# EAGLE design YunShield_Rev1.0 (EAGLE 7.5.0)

## Sheet 1 of 2: MAIN SCHEMATIC
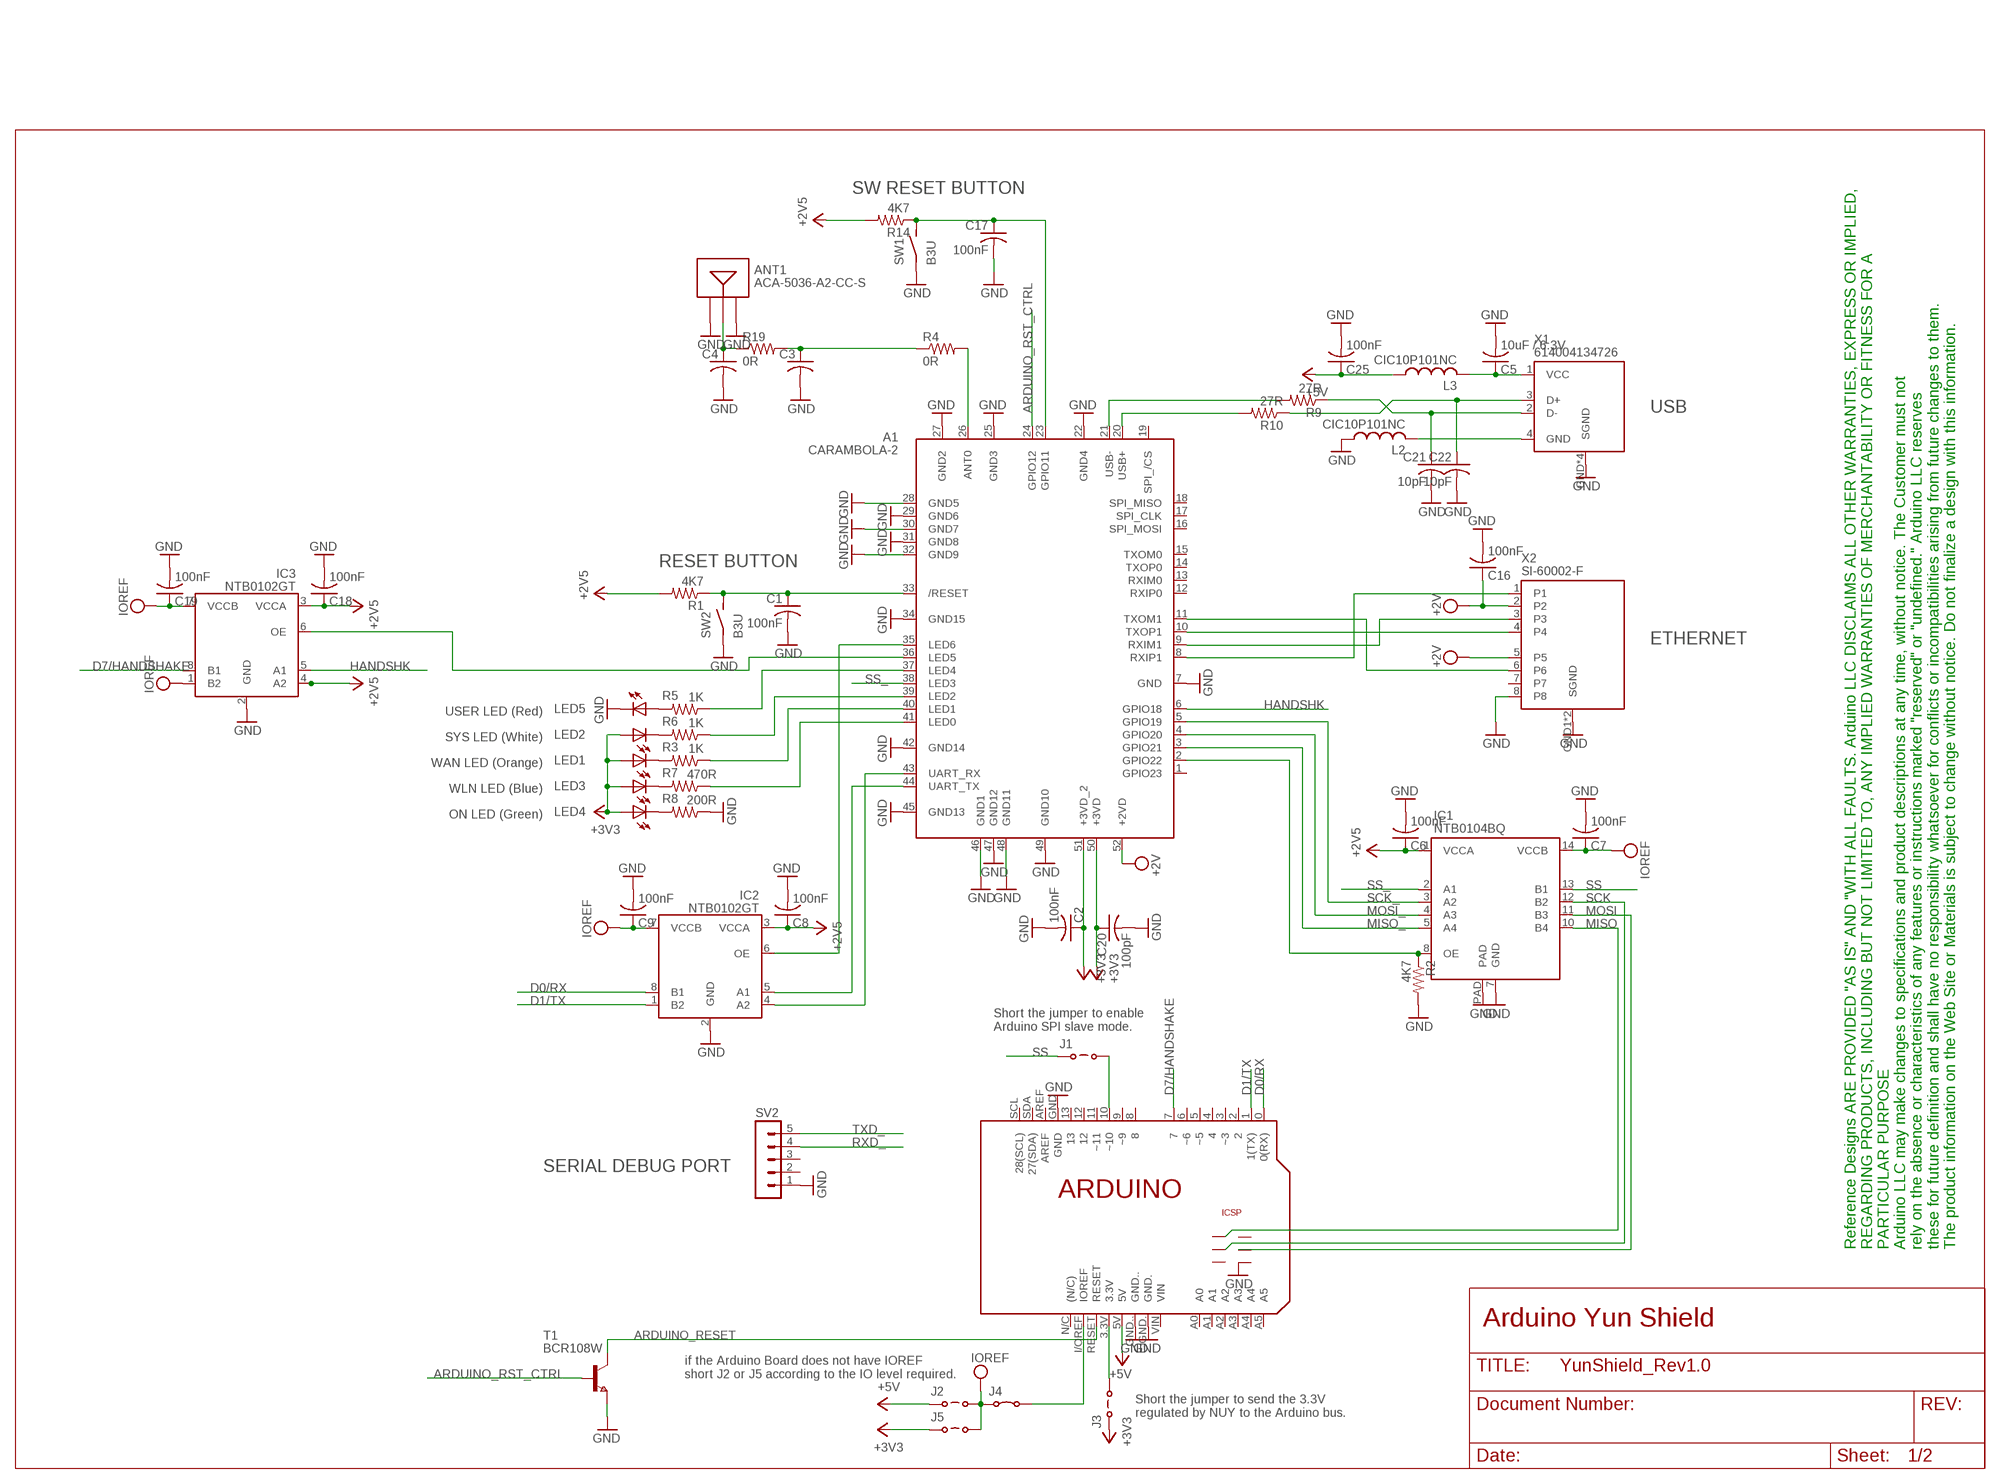
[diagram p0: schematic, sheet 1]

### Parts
A1  CARAMBOLA-2  [CARAMBOLA-2]
ANT1  ACA-5036-A2-CC-S  [ACA-5036-A2-CC-S]
C1  100nF  C-USC0402  [C0402]
C2  100nF  C-USC0402  [C0402]
C3  C-USC0402  [C0402]
C4  C-USC0402  [C0402]
C5  10uF / 6.3V  C-USC1608  [C1608]
C6  100nF  C-USC0402  [C0402]
C7  100nF  C-USC0402  [C0402]
C8  100nF  C-USC0402  [C0402]
C9  100nF  C-USC0402  [C0402]
C16  100nF  C-USC0402  [C0402]
C17  100nF  C-USC0402  [C0402]
C18  100nF  C-USC0402  [C0402]
C19  100nF  C-USC0402  [C0402]
C20  100pF  C-USC0402  [C0402]
C21  10pF  C-USC0402  [C0402]
C22  10pF  C-USC0402  [C0402]
C25  100nF  C-USC0402  [C0402]
IC1  NTB0104BQ  [DHVQFN14]
IC2  NTB0102GT  [XSON8]
IC3  NTB0102GT  [XSON8]
J1  JUMPER-OPEN  [JUMPER-OPEN]
J2  JUMPER-OPEN  [JUMPER-OPEN]
J3  JUMPER-OPEN  [JUMPER-OPEN]
J4  JUMPER-CLOSED  [JUMPER-CLOSED]
J5  JUMPER-OPEN  [JUMPER-OPEN]
L2  CIC10P101NC  L-US  [R0603]
L3  CIC10P101NC  L-US  [R0603]
LED1  LTST-C191KFKT  LEDCHIP-LED0603  [CHIP-LED0603]
LED2  LTW-C193TS5  LEDCHIP-LED0603  [CHIP-LED0603]
LED3  LTST-C191TBKT  LEDCHIP-LED0603  [CHIP-LED0603]
LED4  LTST-C191KGKT  LEDCHIP-LED0603  [CHIP-LED0603]
LED5  LTST-C191KRKT  LEDCHIP-LED0603  [CHIP-LED0603]
PCB1  ARDUINO_UNO  [ARDUINO_UNO]
R1  4K7  R-US_R0402  [R0402]
R2  4K7  R-US_R0402  [R0402]
R3  1K  R-US_R0402  [R0402]
R4  0R  R-US_R0402  [R0402]
R5  1K  R-US_R0402  [R0402]
R6  1K  R-US_R0402  [R0402]
R7  470R  R-US_R0402  [R0402]
R8  200R  R-US_R0402  [R0402]
R9  27R  R-US_R0402  [R0402]
R10  27R  R-US_R0402  [R0402]
R14  4K7  R-US_R0402  [R0402]
R19  0R  R-US_R0402  [R0402]
SV2  MA05-1  [MA05-1]
SW1  B3U  [B3U]
SW2  B3U  [B3U]
T1  BCR108W  NPNSOT323  [SOT323]
X1  614004134726  [614004134726]
X2  SI-60002-F  [SI-60002-F]

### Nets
+3V3: A1.50(+3VD) A1.51(+3VD_2) C2.1 C20.1 J3.1 J5.1 LED1.A LED2.A LED3.A LED4.A ; also sheet 2
+5V: C25.1 J2.1 L3.1 PCB1.5V ; also sheet 2
ARDUINO_RESET: PCB1.RESET T1.1(C)
ARDUINO_RST_CTRL: A1.24(GPIO12) T1.2(B)
D0/RX: IC2.8(B1) PCB1.0(0(RX))
D1/TX: IC2.1(B2) PCB1.1(1(TX))
D7/HANDSHAKE: IC3.8(B1) PCB1.7
GND: A1.7(GND) A1.22(GND4) A1.25(GND3) A1.27(GND2) A1.28(GND5) A1.29(GND6) A1.30(GND7) A1.31(GND8) A1.32(GND9) A1.34(GND15) A1.42(GND14) A1.45(GND13) A1.46(GND1) A1.47(GND12) A1.48(GND11) A1.49(GND10) ANT1.GND ANT1.GND2 C1.2 C2.2 C3.2 C4.2 C5.2 C6.2 C7.2 C8.2 C9.2 C16.2 C17.2 C18.2 C19.2 C20.2 C21.2 C22.2 C25.2 IC1.7(GND) IC1.PAD IC2.2(GND) IC3.2(GND) L2.1 LED5.C PCB1.GND PCB1.GND. PCB1.GND.. PCB1.GND_ R2.2 R8.1 SV2.1 SW1.1 SW2.1 T1.3(E) X1.GND1(SGND) X1.GND2(SGND) X1.GND3(SGND) X1.GND(SGND) X2.8 X2.GND1(SGND) X2.GND2(SGND) ; also sheet 2
HANDSHK: A1.6(GPIO18) IC3.5(A1)
MISO: IC1.10(B4) PCB1.MISO
MISO_: A1.3(GPIO21) IC1.5(A4)
MOSI: IC1.11(B3) PCB1.MOSI
MOSI_: A1.4(GPIO20) IC1.4(A3)
N$1: A1.40(LED1) R3.1
N$2: A1.20(USB+) R10.2
N$3: A1.21(USB-) R9.2
N$4: C5.1 L3.2 X1.1(VCC)
N$5: LED1.C R3.2
N$6: L2.2 X1.4(GND)
N$7: J1.2 PCB1.10(~10)
N$8: J3.2 PCB1.3.3V
N$9: LED5.A R5.2
N$10: C3.1 R4.1 R19.2
N$11: A1.2(GPIO22) IC1.8(OE) R2.1
N$12: A1.37(LED4) R5.1
N$15: LED3.C R7.2
N$16: LED2.C R6.2
N$17: C22.1 R10.1 X1.3(D+)
N$19: A1.23(GPIO11) C17.1 R14.1 SW1.2
N$21: A1.39(LED2) R6.1
N$24: LED4.C R8.2
N$25: A1.41(LED0) R7.1
N$26: A1.35(LED6) IC2.6(OE)
N$27: C21.1 R9.1 X1.2(D-)
N$28: J4.2 PCB1.I/OREF(IOREF)
N$31: A1.36(LED5) IC3.6(OE)
N$33: ANT1.FEED C4.1 R19.1
N$35: A1.26(ANT0) R4.2
N$36: A1.11(TXOM1) X2.6
N$37: A1.10(TXOP1) X2.4
N$38: A1.9(RXIM1) X2.3
N$39: A1.8(RXIP1) X2.1
RESET: A1.33(/RESET) C1.1 R1.1 SW2.2
RXD_: A1.43(UART_RX) IC2.4(A2) SV2.4
SCK: IC1.12(B2) PCB1.SCK
SCK_: A1.5(GPIO19) IC1.3(A2)
SS: IC1.13(B1) J1.1
SS_: A1.38(LED3) IC1.2(A1)
TXD_: A1.44(UART_TX) IC2.5(A1) SV2.5
V+: C6.1 C8.1 C18.1 IC1.1(VCCA) IC2.3(VCCA) IC3.3(VCCA) IC3.4(A2) R1.2 R14.2 ; supply symbol labelled +2V5 ; also sheet 2
VEE: A1.52(+2VD) C16.1 X2.2 X2.5 ; supply symbol labelled +2V
VPP: C7.1 C9.1 C19.1 IC1.14(VCCB) IC2.7(VCCB) IC3.1(B2) IC3.7(VCCB) J2.2 J4.1 J5.2 ; supply symbol labelled IOREF
Unconnected: A1.1(GPIO23) A1.12(RXIP0) A1.13(RXIM0) A1.14(TXOP0) A1.15(TXOM0) A1.16(SPI_MOSI) A1.17(SPI_CLK) A1.18(SPI_MISO) A1.19(SPI_/CS) PCB1.2 PCB1.3(~3) PCB1.4 PCB1.5(~5) PCB1.6(~6) PCB1.8 PCB1.9(~9) PCB1.11(~11) PCB1.12 PCB1.13 PCB1.+5V PCB1.A0 PCB1.A1 PCB1.A2 PCB1.A3 PCB1.A4 PCB1.A5 PCB1.AREF PCB1.N/C((N/C)) PCB1.RESET. PCB1.SCL(28(SCL)) PCB1.SDA(27(SDA)) PCB1.VIN SV2.2 SV2.3 X2.7

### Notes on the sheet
- SW RESET BUTTON
- USB
- RESET BUTTON
- ETHERNET
- USER LED (Red)
- SYS LED (White)
- WAN LED (Orange)
- WLN LED (Blue)
- ON LED (Green)
- Short the jumper to enable
  Arduino SPI slave mode.
- SERIAL DEBUG PORT
- Reference Designs ARE PROVIDED "AS IS" AND "WITH ALL FAULTS. Arduino LLC DISCLAIMS ALL OTHER WARRANTIES, EXPRESS OR IMPLIED,
  REGARDING PRODUCTS, INCLUDING BUT NOT LIMITED TO, ANY IMPLIED WARRANTIES OF MERCHANTABILITY OR FITNESS FOR A 
  PARTICULAR PURPOSE 
  Arduino LLC may make changes to specifications and product descriptions at any time, without notice. The Customer must not
  rely on the absence or characteristics of any features or instructions marked "reserved" or "undefined." Arduino LLC reserves
  these for future definition and shall have no responsibility whatsoever for conflicts or incompatibilities arising from future changes to them.
  The product information on the Web Site or Materials is subject to change without notice. Do not finalize a design with this information.
- Arduino Yun Shield
- if the Arduino Board does not have IOREF
  short J2 or J5 according to the IO level required.
- Short the jumper to send the 3.3V 
  regulated by NUY to the Arduino bus.

## Sheet 2 of 2: SWITCH-MODE POWER SUPPLY
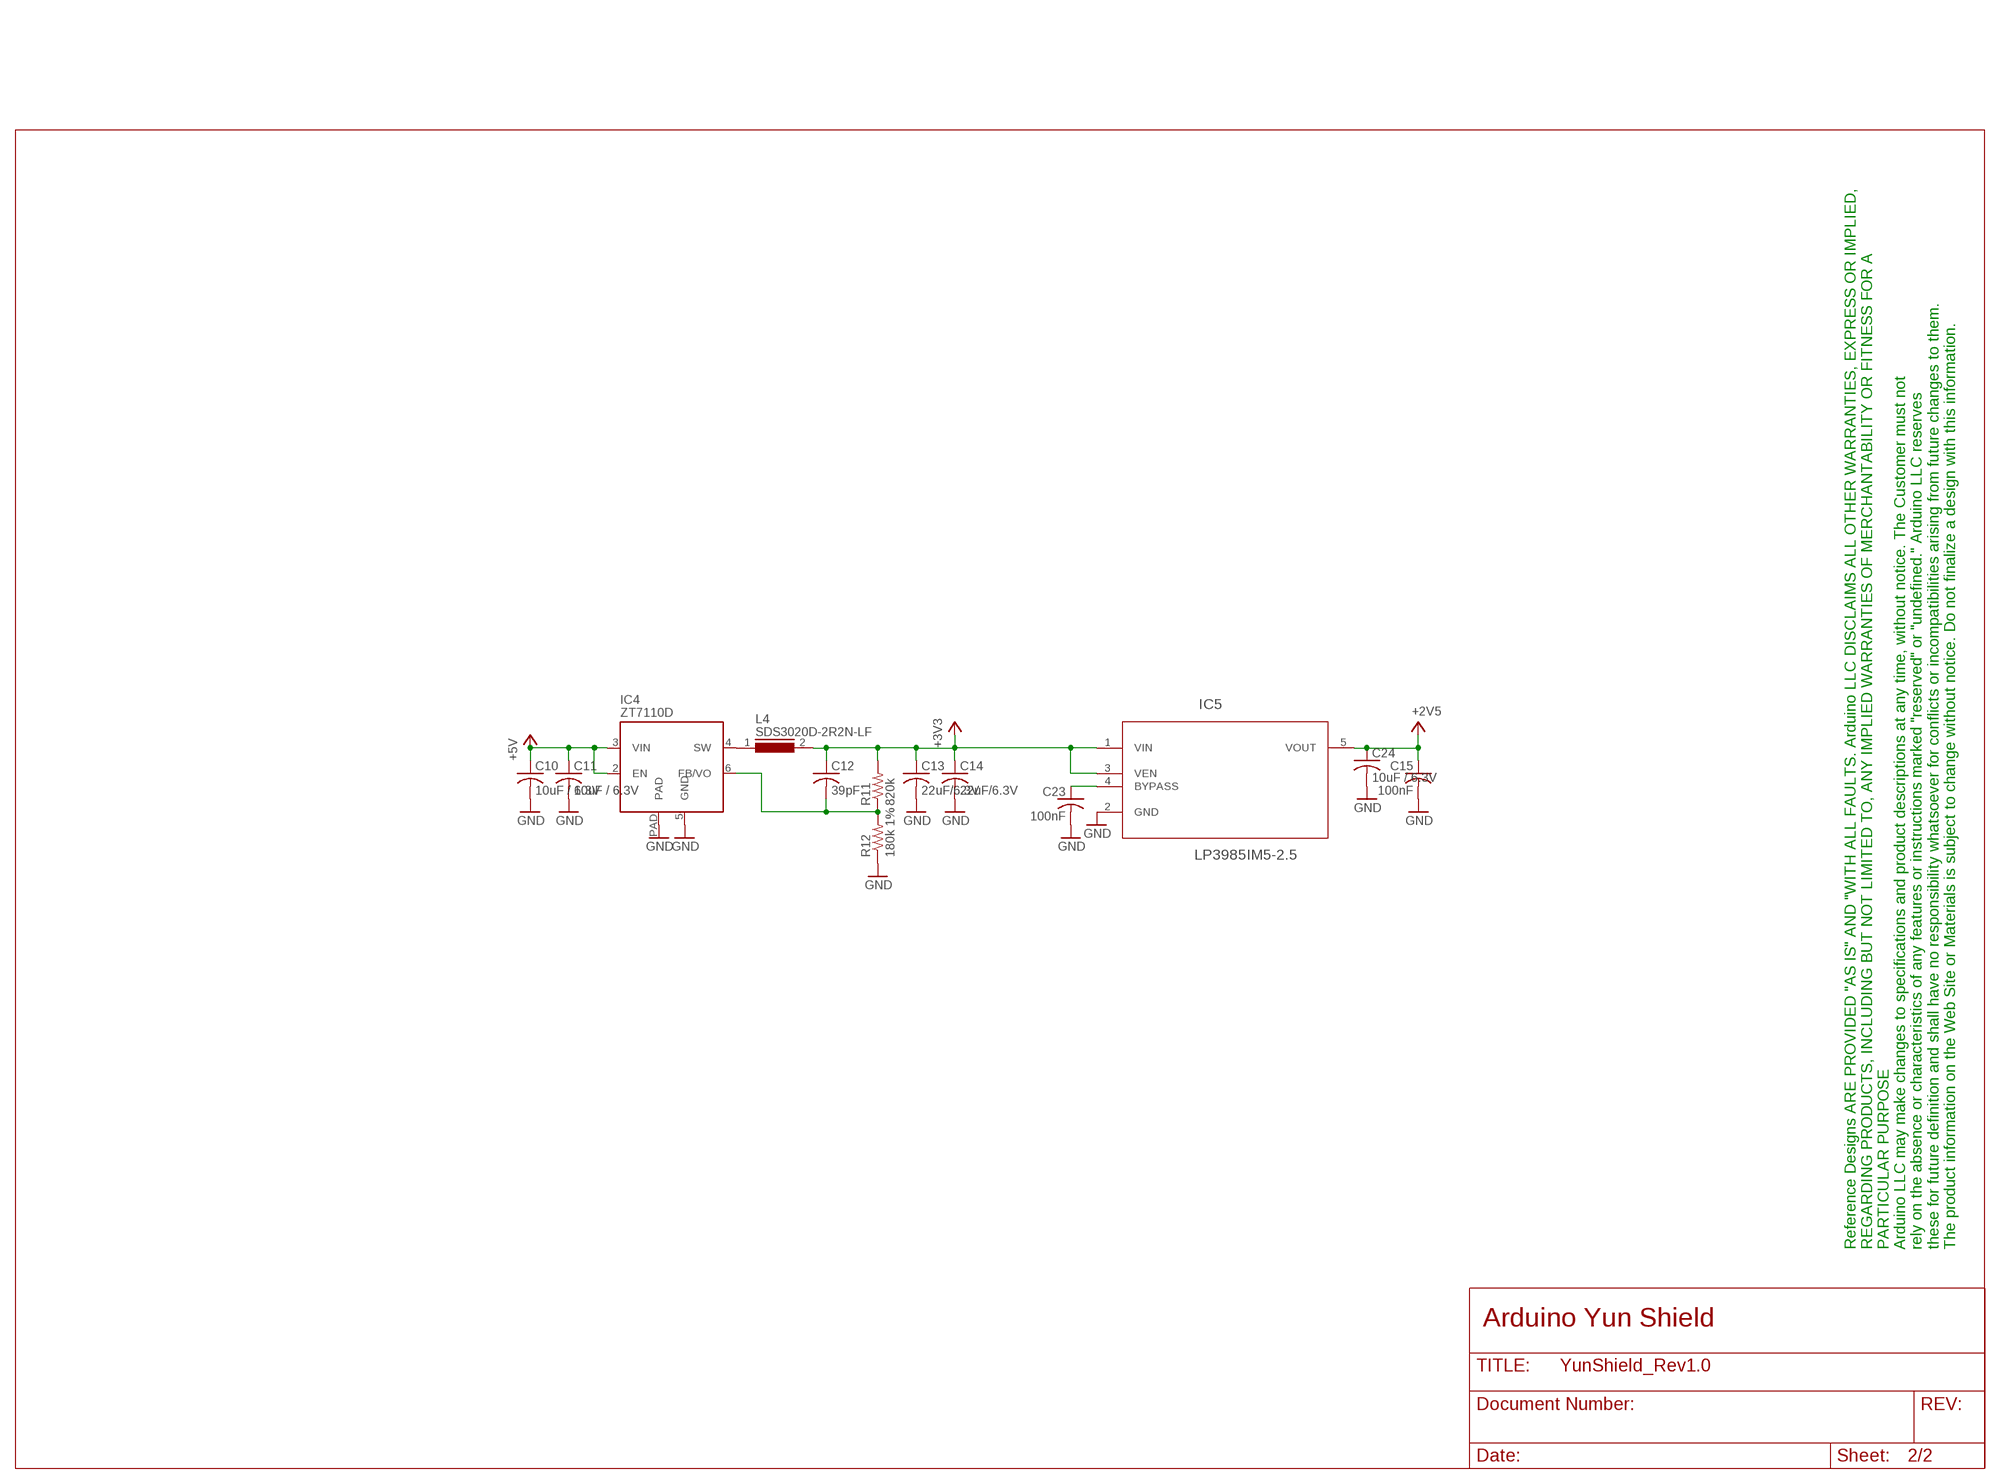
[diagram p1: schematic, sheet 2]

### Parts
C10  10uF / 6.3V  C-USC1608  [C1608]
C11  10uF / 6.3V  C-USC1608  [C1608]
C12  39pF  C-USC0402  [C0402]
C13  22uF/6.3V  C-USC1206  [C1206]
C14  22uF/6.3V  C-USC1206  [C1206]
C15  100nF  C-USC0402  [C0402]
C23  100nF  C-USC0402  [C0402]
C24  10uF / 6.3V  C-USC1608  [C1608]
IC4  ZT7110D  [DFN-6]
IC5  LP3985IM5-2.5  [SOT95P300X120-5N]
L4  SDS3020D-2R2N-LF  [SDS3020D-2R2N-LF]
R11  820k  R-US_R0402  [R0402]
R12  180k 1%  R-US_R0402  [R0402]

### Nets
+3V3: C12.1 C13.1 C14.1 IC5.1(VIN) IC5.3(VEN) L4.2 R11.2 ; also sheet 1
+5V: C10.1 C11.1 IC4.2(EN) IC4.3(VIN) ; also sheet 1
GND: C10.2 C11.2 C13.2 C14.2 C15.2 C23.2 C24.2 IC4.5(GND) IC4.PAD IC5.2(GND) R12.1 ; also sheet 1
N$18: C12.2 IC4.6(FB/VO) R11.1 R12.2
N$20: IC4.4(SW) L4.1
RESET2: C23.1 IC5.4(BYPASS)
V+: C15.1 C24.1 IC5.5(VOUT) ; supply symbol labelled +2V5 ; also sheet 1

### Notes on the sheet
- Reference Designs ARE PROVIDED "AS IS" AND "WITH ALL FAULTS. Arduino LLC DISCLAIMS ALL OTHER WARRANTIES, EXPRESS OR IMPLIED,
  REGARDING PRODUCTS, INCLUDING BUT NOT LIMITED TO, ANY IMPLIED WARRANTIES OF MERCHANTABILITY OR FITNESS FOR A 
  PARTICULAR PURPOSE 
  Arduino LLC may make changes to specifications and product descriptions at any time, without notice. The Customer must not
  rely on the absence or characteristics of any features or instructions marked "reserved" or "undefined." Arduino LLC reserves
  these for future definition and shall have no responsibility whatsoever for conflicts or incompatibilities arising from future changes to them.
  The product information on the Web Site or Materials is subject to change without notice. Do not finalize a design with this information.
- Arduino Yun Shield

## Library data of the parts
A1 = KRB-EX1002-G1413:CARAMBOLA-2
ANT1 = KRB-EX1002-G1413:ACA-5036-A2-CC-S
C1 C3 C4 C6-C9 C15-C19 C21-C23 C25 = KRB-EX1002-G1413:C-US: CAPACITOR, American symbol
C2 C5 C10-C14 C20 C24 = rcl:C-US: CAPACITOR, American symbol
IC1 = KRB-EX1002-G1413:NTB0104
IC2 IC3 = KRB-EX1002-G1413:NTB0102
IC4 = KRB-EX1002-G1413:ZT7110
IC5 = LP3985IM5-2.5:LP3985IM5-2.5: Low-Dropout CMOS Voltage Regulator; MPN: LP3985IM5-25; OC_FARNELL: 1469024; OC_NEWARK: 23K8220; PACKAGE: SOT-5; SIPPLIER: NationalSemiconductor
J1-J3 J5 = rcl:JUMPER-OPEN
J4 = rcl:JUMPER-CLOSED
L2 L3 = rcl:L-US: INDUCTOR, American symbol
L4 = KRB-EX1002-G1413:SDS3020D-2R2N-LF
LED1-LED5 = led:LED: LED
PCB1 = KRB-EX1002-G1413:ARDUINO_UNO: Device for representing an Arduino Uno board with a footprint in an EAGLE design. Created by Dave Young for Element14. More EAGLE documentation at: http://www.element14.com/community/community/knode/cadsoft_eagle
R1-R3 R5-R12 R14 = rcl:R-US_: RESISTOR, American symbol
R4 R19 = KRB-EX1001-G1405:R-US_: RESISTOR, American symbol
SV2 = con-lstb:MA05-1: PIN HEADER; OC_FARNELL: unknown; OC_NEWARK: unknown
SW1 SW2 = 8DEV-1100-0001:B3U
T1 = zetex:NPNSOT323: NPN TRANSISTOR; MPN: DSS4160U-7; OC_FARNELL: 1710696; OC_NEWARK: 25R4558
X1 = KRB-EX1002-G1413:614004134726
X2 = KRB-EX1002-G1413:SI-60002-F

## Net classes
1 power: width 0.254 mm, drill 0.61 mm, clearance 0.254 mm
2 gnd: width 0.254 mm, drill 0.61 mm, clearance 0.254 mm
3 usbvcc: width 0.254 mm, drill 0.61 mm, clearance 0.254 mm
4 aref: width 0.254 mm, drill 0.61 mm, clearance 0.254 mm

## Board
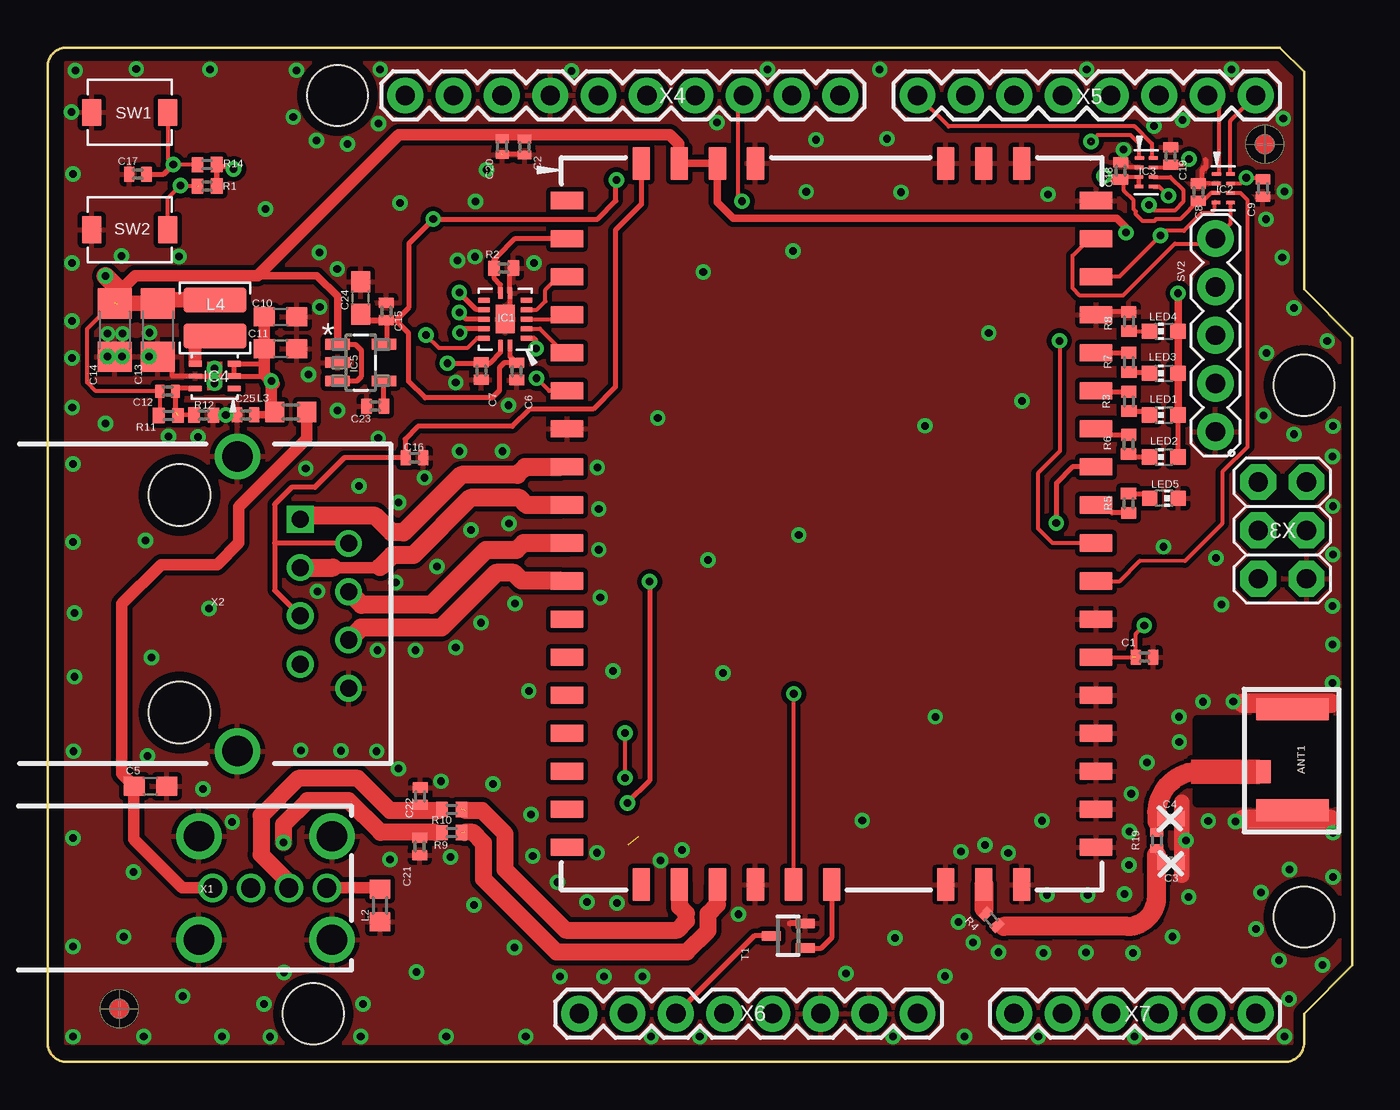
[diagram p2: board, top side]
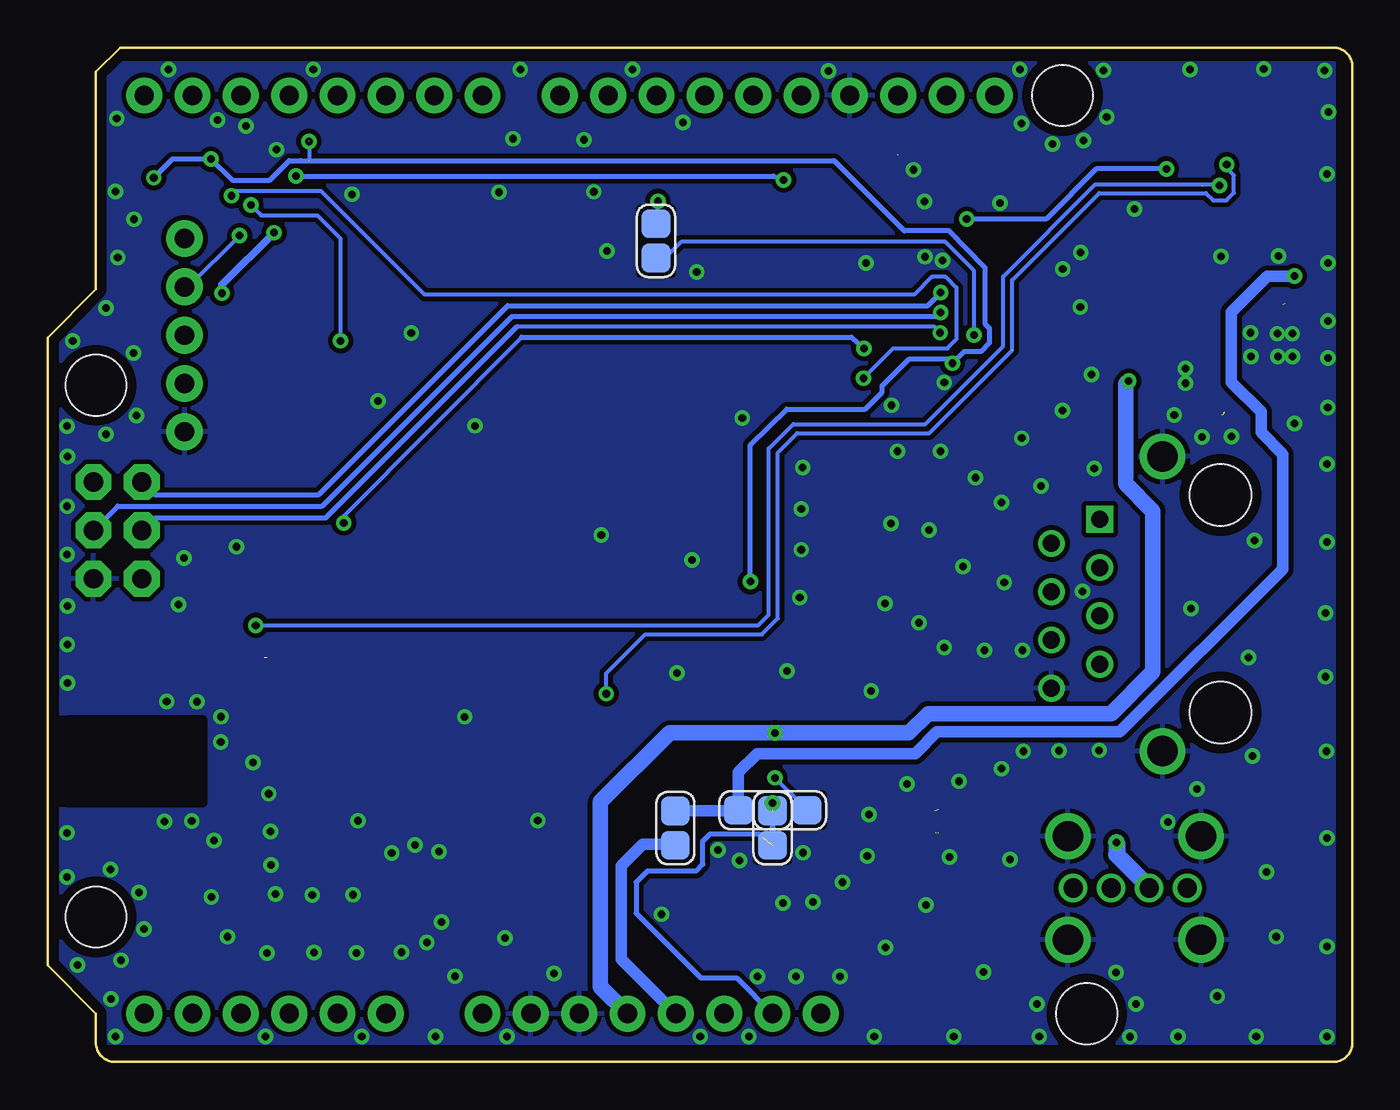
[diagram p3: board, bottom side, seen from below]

Size 68.58 x 53.31 mm. Coordinates in mm from the lower left corner, seen from the top.
Copper layers (1*16): Top 0.035mm / dielectric 1mm / Bottom 0.035mm
Design rules "default *": minimum track width 4mil, minimum drill 0.39mm, track to track 4mil, track to pad 4mil, pad to pad 4mil, via to via 4mil, smd to smd 4mil, copper to edge 20mil, drill to drill 0.5mm, minimum pad ring 10mil, minimum via ring 8mil, stop-mask expansion 2mil, vias tented up to drill 0.55mm, thermal gap 10mil
tRestrict: area 60.4,13.6 to 67.5,18; area 62.8,13.6 to 68.5,18
bRestrict: area 60.4,13.6 to 67.5,18; area 62.8,13.6 to 68.5,18

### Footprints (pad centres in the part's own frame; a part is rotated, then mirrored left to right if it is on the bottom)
CARAMBOLA-2 = smd 0.9 x 1.7: 1 -17.05,-12.8; 2 -15.05,-12.8; 3 -13.05,-12.8; 4 -11.05,-12.8; 5 -9.05,-12.8; 6 -7.05,-12.8; 7 -5.05,-12.8; 8 -3.05,-12.8; 9 -1.05,-12.8; 10 0.95,-12.8; 11 2.95,-12.8; 12 4.95,-12.8; 13 6.95,-12.8; 14 8.95,-12.8; 15 10.95,-12.8; 16 12.95,-12.8; 17 14.95,-12.8; 18 16.95,-12.8; 28 16.95,15; 29 14.95,15; 30 12.95,15; 31 10.95,15; 32 8.95,15; 33 6.95,15; 34 4.95,15; 35 2.95,15; 36 0.95,15; 37 -1.05,15; 38 -3.05,15; 39 -5.05,15; 40 -7.05,15; 41 -9.05,15; 42 -11.05,15; 43 -13.05,15; 44 -15.05,15; 45 -17.05,15 | smd 1.7 x 0.9: 19 18.9,-8.9; 20 18.9,-6.9; 21 18.9,-4.9; 22 18.9,-2.9; 23 18.9,-0.9; 24 18.9,1.1; 25 18.9,7.1; 26 18.9,9.1; 27 18.9,11.1; 46 -19,11.1; 47 -19,9.1; 48 -19,7.1; 49 -19,-2.9; 50 -19,-4.9; 51 -19,-6.9; 52 -19,-8.9
ACA-5036-A2-CC-S = smd 0.75 x 1.2: FEED 1.525,0.632 | smd 3.8 x 1.15: GND 0,2.658; GND2 0,-2.658
C0402 = smd 0.533 x 0.787: 1 -0.457,0; 2 0.457,0
C0402' = smd 0.457 x 0.686: 1 -0.419,0; 2 0.419,0
C1608 = smd 1.1 x 1: 1 -0.85,0; 2 0.85,0
C1206 = smd 1.6 x 1.8: 1 -1.4,0; 2 1.4,0
DHVQFN14 = smd 0.6 x 0.25: 1 -1.375,-0.25; 7 1.375,-0.25; 8 1.375,0.25; 14 -1.375,0.25 | smd 0.25 x 0.6: 2 -1,-1.125; 3 -0.5,-1.125; 4 0,-1.125; 5 0.5,-1.125; 6 1,-1.125; 9 1,1.125; 10 0.5,1.125; 11 0,1.125; 12 -0.5,1.125; 13 -1,1.125 | smd 1.5 x 1: PAD 0,0
XSON8 = smd 0.2 x 0.5: 1 -0.75,-0.35 | smd 0.2 x 0.45: 2 -0.25,-0.375; 3 0.25,-0.375; 4 0.75,-0.375; 5 0.75,0.375; 6 0.25,0.375; 7 -0.25,0.375; 8 -0.75,0.375
DFN-6 = smd 0.3 x 0.7: 1 -0.65,-1.025; 2 0,-1.025; 3 0.65,-1.025; 4 0.65,1.025; 6 -0.65,1.025 | smd 0.25 x 0.7: 5 0,1.025 | smd 1.27 x 0.508: PAD 0,0
SOT95P300X120-5N = smd 1.27 x 0.559: 1 -1.219,0.965; 2 -1.219,0; 3 -1.219,-0.965; 4 1.219,-0.965; 5 1.219,0.965
JUMPER-OPEN = smd 1.5 x 1.5: 1 -0.9,0; 2 0.9,0
JUMPER-CLOSED = smd 1.5 x 1.5: 1 -0.9,0; 2 0.9,0
R0603 = smd 1 x 1.1: 1 -0.85,0; 2 0.85,0
SDS3020D-2R2N-LF = smd 1.3 x 3.3: 1 -0.95,0; 2 0.95,0
CHIP-LED0603 = smd 0.8 x 0.8: A 0,-0.75; C 0,0.75
ARDUINO_UNO = drill 1.016 pad 1.88: 0 63.5,50.8; 1 60.96,50.8; 2 58.42,50.8; 3 55.88,50.8; 3.3V 35.56,2.54; 4 53.34,50.8; 5 50.8,50.8; 5V 38.1,2.54; 6 48.26,50.8; 7 45.72,50.8; 8 41.656,50.8; 9 39.116,50.8; 10 36.576,50.8; 11 34.036,50.8; 12 31.496,50.8; 13 28.956,50.8; A0 50.8,2.54; A1 53.34,2.54; A2 55.88,2.54; A3 58.42,2.54; A4 60.96,2.54; A5 63.5,2.54; AREF 23.876,50.8; GND 26.416,50.8; GND. 43.18,2.54; GND.. 40.64,2.54; I/OREF 30.48,2.54; N/C 27.94,2.54; RESET 33.02,2.54; SCL 18.796,50.8; SDA 21.336,50.8; VIN 45.72,2.54 | drill 1.016 pad 1.88 octagon: +5V 66.167,30.48; GND_ 66.167,25.4; MISO 63.627,30.48; MOSI 66.167,27.94; RESET. 63.627,25.4; SCK 63.627,27.94 | hole 3.2: 66.04,7.62; 66.04,35.56; 15.24,50.8; 13.97,2.54
R0402 = smd 0.61 x 0.787: 1 -0.508,0 | smd 0.61 x 0.813: 2 0.508,0
R0402' = smd 0.457 x 0.686: 1 -0.419,0; 2 0.419,0
MA05-1 = drill 1.016 pad 1.93: 1 -5.08,0; 2 -2.54,0; 3 0,0; 4 2.54,0; 5 5.08,0
B3U = smd 1 x 1.4: 1 -2,0; 2 2,0
SOT323 = smd 0.5 x 1: 1 0,0.9; 2 -0.65,-0.9; 3 0.65,-0.9
614004134726 = drill 1: 1 0,-6; 2 0,-4; 3 0,-2; 4 0,0 | drill 1.6: GND -2.72,0.27; GND1 2.72,0.27; GND2 -2.72,-6.73; GND3 2.72,-6.73
SI-60002-F = drill 0.9 square: 1 -4.445,6.35 | drill 0.9: 2 -3.175,8.89; 3 -1.905,6.35; 4 -0.635,8.89; 5 0.635,6.35; 6 1.905,8.89; 7 3.175,6.35; 8 4.445,8.89 | drill 1.6: GND1 -7.745,3.05; GND2 7.745,3.05 | hole 3.25: -5.715,0; 5.715,0

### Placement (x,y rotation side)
A1  40.11,28.23 270 top
ANT1  65.42,15.88 180 top
C1  57.65,21.28 0 top
C2  100nF  [C0402']  25.07,48.09 270 top
C3  59.05,10.5 0 top
C4  59.04,12.78 0 top
C5  5.41,14.5 0 top
C6  24.65,36.3 270 top
C7  22.81,36.32 270 top
C8  60.48,45.71 90 top
C9  63.88,45.93 270 top
C10  12.25,39.17 0 top
C11  12.25,37.49 0 top
C12  39pF  [C0402']  6.31,35.26 0 top
C13  5.79,38.47 270 top
C14  3.53,38.47 270 top
C15  17.81,39.45 90 top
C16  19.28,31.76 0 top
C17  4.74,46.66 180 top
C18  56.39,46.84 90 top
C19  59.03,47.61 90 top
C20  100pF  [C0402']  23.89,48.11 270 top
C21  19.55,11.33 270 top
C22  19.58,13.97 90 top
C23  17.22,34.47 180 top
C24  16.46,40.16 90 top
C25  10.41,34.01 180 top
IC1  24.05,39.04 90 top
IC2  61.79,45.92 270 top
IC3  57.74,46.76 270 top
IC4  8.79,36.05 90 top
IC5  16.46,36.75 0 top
J1  36.6,43.15 90 bottom
J2  29.57,13.23 180 bottom
J3  35.59,12.29 270 bottom
J4  30.48,12.29 270 bottom
J5  31.37,13.23 0 bottom
L2  17.47,8.22 90 top
L3  12.78,34.16 0 top
L4  8.79,39.1 90 top
LED1  58.67,34 90 top
LED2  58.67,31.8 90 top
LED3  58.67,36.2 90 top
LED4  58.67,38.4 90 top
LED5  58.68,29.63 270 top
PCB1  0,0 0 top
R1  8.38,46.03 0 top
R2  23.97,41.72 0 top
R3  56.83,34.72 270 top
R4  0R  [R0402']  49.6,7.47 135 top
R5  56.82,29.36 90 top
R6  56.82,32.46 270 top
R7  56.83,36.77 270 top
R8  56.83,38.92 270 top
R9  21.24,12.06 0 top
R10  21.24,13.27 0 top
R11  6.35,33.98 180 top
R12  8.21,33.99 180 top
R14  8.38,47.17 0 top
R19  0R  [R0402']  58.3,11.64 270 top
SV2  61.38,38.2 90 top
SW1  4.32,49.91 0 top
SW2  4.32,43.74 0 top
T1  38.93,6.63 90 top
U$12  [FIDUCIAL_G10]  3.77,2.8 0 top
U$13  [FIDUCIAL_G10]  63.98,48.22 0 top
X1  14.68,9.14 270 top
X2  6.93,24.08 270 top

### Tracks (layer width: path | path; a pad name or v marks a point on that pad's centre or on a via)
+3V3  (via drill 0.4)  (1 unrouted)
  Top 0.2: R11.2 5.89,34.02 C12.1 2.53,35.26 2.08,35.71 2.08,38.53 2.72,39.17 2.83,39.17 C14.1 | 8.89,41.27 8.89,41.33 8.87,41.33
  Top 0.254: 35.32,47.34 A1.50 | 3.67,40.39 3.67,40.01 | 33.25,47.18 A1.51 | 22.76,48.72 22.77,48.74 | 23.89,48.72 23.9,48.74 | C2.1 25.07,48.72 25.04,48.74 | C20.1 23.89,48.71 23.85,48.74 | LED2.A LED1.A | IC5.1 16.18,37.72 16.48,37.41 16.48,36.02 16.26,35.79 IC5.3
  Top 0.406: 33.17,47.19 A1.51 A1.50 35.21,45.17 36.03,44.35 56.19,44.35 56.67,43.86 v56.67,43.59 | LED1.A LED3.A LED4.A 59.42,39.59 v59.42,40.4 | 3.5,39.84 C14.1 | IC5.1 15.24,40.23 14.15,41.33 10.97,41.33
  Top 0.61: 3.67,39.83 3.67,40.39 4.61,41.33 8.87,41.33 10.97,41.33 11.05,41.33 18.46,48.74 22.77,48.74 23.85,48.74 23.9,48.74 25.04,48.74 32.7,48.74 33.17,48.26 33.17,47.34 33.17,47.33 | 3.67,39.83 3.67,39.7 | 33.17,47.19 33.17,47.33 | 33.17,47.33 33.17,47.68 | 3.76,39.92 3.67,39.83
  Top 0.813: L4.2 5.98,40.05 C13.1 3.81,39.87 3.76,39.92
  Top 0.95: v3.05,41.3 3.67,40.68 3.67,39.7
  Bottom 0.406: v59.42,40.4 59.42,40.84 v56.67,43.59
  Bottom 0.61: J3.1 32.31,13.19 J5.1 32.27,15.23 31.29,16.2 22.99,16.2 21.84,17.35 12.22,17.35 3.66,25.91 3.66,31.95 4.8,33.1 4.8,34.16 6.38,35.71 6.38,39.4 4.47,41.3 v3.05,41.3
+5V  (via drill 0.4)
  Top 0.2: v30.35,14.94 v30.35,17.3
  Top 0.254: 11.38,36.12 11.39,36.05 IC4.2 IC4.3 9.71,36.7 9.7,36.71 | 11.38,36.12 11.37,36.21 | 9.63,36.71 9.7,36.71 | 9.7,36.71 11.23,36.71 | 11.39,36.15 11.39,36.13 11.38,36.12
  Top 0.406: C25.1 11.93,34.01 L3.1
  Top 0.606: C11.1 11.39,36.15
  Top 0.61: C11.1 C10.1 | 11.39,36.15 v11.76,35.79 | 11.9,35.65 v11.76,35.79 | L3.1 11.76,34.33 v11.76,35.79
  Bottom 0.2: J2.1 28.67,13.25 v30.35,14.94
  Bottom 0.813: PCB1.5V 39.52,3.96 39.52,13.66 35.89,17.3 v30.35,17.3 23.32,17.3 22.3,18.31 12.68,18.31 10.49,20.5 10.49,28.96 11.91,30.38 11.91,35.64 v11.76,35.79
ARDUINO_RESET
  Top 0.254: T1.1 37.15,6.63 33.57,3.05 PCB1.RESET
ARDUINO_RST_CTRL
  Top 0.254: T1.2 40.67,5.98 41.21,6.52 A1.24
D0/RX
  Top 0.2: IC2.8 62.17,49.47 PCB1.0
D1/TX
  Top 0.2: IC2.1 61.59,46.67 61.59,50.17 PCB1.1
D7/HANDSHAKE
  Top 0.2: 57.13,49.17 58.04,48.26 58.04,47.51 IC3.8
  Top 0.203: 57.13,49.17 47.35,49.17 PCB1.7
GND  (via drill 0.4, 0.4 pad 0.3)  (1 unrouted)
  Top 0.2: 56.51,47.16 C18.2 56.66,47.01 IC3.2 | 61.09,46.17 60.7,46.17
  Top 0.254: IC4.PAD IC4.5 6.56,36.05 6.56,37.08 5.79,37.08 C13.2 | IC1.PAD 24.16,39.14 24.16,39.22 24.3,39.37 IC1.7 24.3,41.48 R2.2 | 60.87,47.42 60.87,46.96 | 60.7,46.17 60.69,46.17 60.69,46.82 60.8,47.05 | R8.1 55.26,39.43 A1.42 | 25.07,47.7 23.88,47.7
  Top 0.305: T1.3 39.03,7.28
  Top 0.813: 59.62,13.66 59.62,9.82
  Top 1.016: 62.86,12.74 67.38,12.74 | 62.84,18.86 67.44,18.86
  other vias: 39.48,27.7 61.42,26.49 42.82,12.68 48.01,11.05 13.71,36.12 3.14,37.08 3.92,37.08 5.32,37.08 24.22,34.52 67.26,37.9 62.22,52.17 47.87,7.35 48.65,6.27 49.98,5.77 52.34,5.74 54.57,5.75 50.49,10.98 49.26,11.41 52.52,8.79 54.67,8.78 56.95,14.1 57.04,5.72 59.13,6.58 59.83,11.64 59.97,8.66 21.18,10.76 16.46,1.33 8.78,36.45 3.88,42.37 4.51,9.98 44.53,6.52 29.24,4.49 22.46,42.32 32.07,33.84 21.45,35.7 25.56,41.99 59.46,18.14 46.11,33.43 39.18,42.63 34.46,41.53 1.33,1.33 1.34,27.32 16.36,30.27 1.29,41.99 62.32,18.95 64.89,42.28 18.52,45.15 1.29,36.99 56.83,10.34 1.28,38.95 67.53,19.91 67.53,23.96 67.55,9.73 63.52,6.98 46.66,18.14 67.55,33.42 49.47,38.31 56.55,47.95 44.85,45.71 25.13,1.33 1.34,31.44 5.37,38.33 3.95,38.28 3.16,38.28 56.86,12.12 9.36,34 57.78,15.74 59.48,16.81 64.73,5.34 1.34,6.08 1.34,11.77 44.12,48.52 40.39,48.47 52.58,45.6 58.66,27.08 39.88,45.73 35.19,49.37 6.91,42.34 9.17,1.33 67.54,21.93 60.73,18.93 61,12.66 65.28,10.12 52.27,12.68 61.7,24.04 67,5.1 67.53,31.82 13.09,52.12 1.34,46.67 43.73,52.16 63.78,8.9 1.26,49.93 36.31,7.76 8.78,35.67 20.95,1.34 47.16,4.51 41.96,4.65 65.5,32.99 58.14,49.2 59.66,49.5 64.04,44.29 65.51,39.64 54.62,52.16 64.06,37.27 1.3,34.39 4.66,52.19 15.76,48.24 27.54,52.09 17.48,52.16 37.85,52.17 57.12,1.34 52.07,1.33 65,1.33 44.43,1.34 34.27,1.34 31.72,1.34 23.07,46.89 22.49,45.22 51.21,34.74 64.94,49.59 48.19,1.34 67.56,12.04 3.05,33.56 12.91,49.66 17.38,49.32 8.54,52.16 5.05,1.34 11.7,1.33 11.38,3.05 12.42,4.71 16.58,3.05 67.55,26.67 67.55,29.21 63.9,33.97 65.24,3.3 65.02,45.75 11.45,44.83 56.6,8.83 62.43,12.64 19.4,4.72 14.14,48.43 28.87,10.99 31.27,4.49 18.3,25.19 20.46,26.03 28.89,31.24 24.24,28.29 22.26,27.96 17.34,21.64 19.34,21.64 21.45,21.79 22.78,23.09 24.57,24.1 23.91,32.1 21.65,32.1 19.82,30.7 18.45,29.41 14.19,24.74 28.97,29.05 28.97,26.92 24.54,6.02 26.92,4.49 22.4,8.25 29.92,8.35 28.35,8.4 26.8,9.45 25.5,10.82 25.4,13 23.42,14.6 20.68,14.75 18.44,15.41 17.3,16.33 15.42,16.35 13.31,16.38 18,10.64 9.7,12.62 4.01,6.58 1.36,16.33 1.41,20.24 8.17,14.35 1.41,23.6 1.46,52.11 5.45,21.26 8.48,23.83 5.15,27.41 5.25,16.08 7.1,3.46 32.22,10.59 33.34,11.15 7.9,32.85 6.35,32.87 14.31,39.67 29.73,20.55 35.49,20.44 25.29,19.51 34.7,26.39 15.24,34.23 29.05,24.41 21.54,42.11 17.38,32.78 13.57,31.18 15.22,41.68 14.28,42.54
  pour Top (isolate 0.254): 1,52.5 68,52.5 68,1 1,1
  pour Bottom (isolate 0.254): 68,52.5 1,52.5 1,1 68,1
HANDSHK  (via drill 0.4)
  Top 0.2: IC3.5 58.42,46.01 v58.91,45.52
  Top 0.203: A1.6 26.36,35.28 v25.7,35.94
  Bottom 0.2: v58.91,45.52 58.66,45.77 54.2,45.77 48.76,40.33 23.04,40.33 22.11,41.27 21.38,41.27 | 24.12,37.51 21.29,37.51 20.82,37.99
  Bottom 0.203: 21.38,41.27 20.82,40.7 20.82,37.99 | 24.12,37.51 v25.7,35.94
MISO  (via drill 0.4)
  Top 0.254: IC1.10 22.54,39.54 v21.64,40.44
  Bottom 0.254: PCB1.MISO 63.6,30.48 62.94,29.82 54.33,29.82 44.4,39.75 22.33,39.75 v21.64,40.44
MISO_
  Top 0.203: IC1.5 25.72,39.54 26.16,39.98 26.16,40.59 26.85,41.27 A1.3
MOSI  (via drill 0.4)
  Top 0.254: IC1.11 22,39.04 v21.64,39.4
  Bottom 0.254: PCB1.MOSI 64.9,29.21 54.15,29.21 44.17,39.19 21.84,39.19 v21.64,39.4
MOSI_
  Top 0.203: A1.4 27.25,39.33 26.96,39.04 IC1.4
N$1
  Top 0.254: A1.40 55.16,35.22 R3.1
N$2  (1 unrouted)
  Top 0.203: 33.2,9.32 A1.20
  Top 0.9: 21.97,13.21 22.84,13.21 24.05,11.99 24.05,10.11 27.23,6.93 33.1,6.93 33.58,7.42 33.58,7.8 33.22,8.15 33.22,9.31 A1.20
N$3  (1 unrouted)
  Top 0.254: 35.16,9.37 A1.21
  Top 0.406: 21.76,12.04 R9.2
  Top 0.9: 21.92,12.06 22.35,12.06 22.91,11.51 22.91,9.63 26.75,5.79 33.6,5.79 34.72,6.91 34.72,7.8 35.2,8.28 A1.21
N$4
  Top 0.61: 4.52,14.53 3.91,15.14 3.91,24.08 5.97,26.14 8.91,26.14 10.06,27.28 10.06,29.18 13.63,32.76 L3.2 | 4.52,14.53 C5.1 | X1.1 7.09,9.14 4.52,11.71 4.52,14.53
N$5
  Top 0.254: R3.2 57.71,34.21 LED1.C
N$6
  Top 0.61: X1.4 17.44,9.14 L2.2
N$7  (via drill 0.4)
  Top 0.2: PCB1.10 36.27,50.49 36.27,45.47 v36.5,45.24
  Bottom 0.2: J1.2 36.5,44.45 v36.5,45.24
N$8
  Bottom 0.61: PCB1.3.3V 38.43,5.41 38.43,10.31 37.29,11.46 35.73,11.46 J3.2
N$9
  Top 0.254: R5.2 57.93,29.87 LED5.A
N$10
  Top 0.254: R19.2 58.3,10.88 | 58.3,10.88 58.29,10.88 | C3.1 58.59,10.6 58.3,10.88 | R4.1 50.2,7.18 50.26,7.12
  Top 1: 50.26,7.12 56.76,7.12 arc90 58.29,8.73 58.29,10.88
N$11
  Top 0.254: A1.2 27.29,43.26 27.25,43.26 27.23,43.28 24.59,43.28 23.62,42.32 23.47,42.16 R2.1 23.48,41.18 23.8,40.85 IC1.8
N$12
  Top 0.254: R5.1 55.96,28.85 55.55,29.26 55.12,29.26 A1.37
N$15
  Top 0.254: R7.2 57.86,36.26 LED3.C
N$16
  Top 0.254: R6.2 56.97,31.8 LED2.C
N$17
  Top 0.254: C22.1 19.82,13.27 R10.1 20.56,13.27 20.6,13.21
  Top 0.9: 20.6,13.21 18.01,13.21 16.31,14.91 13.18,14.91 11.23,12.95 11.23,10.9 12.68,9.45 12.68,9.15 X1.3
N$18  (2 unrouted)
  Top 0.254: 6.74,34.15 C12.2 6.68,35.31 6.68,35.33 6.73,35.33 6.82,35.4 IC4.6 | R12.2 6.82,34.01
N$19  (via drill 0.4)  (1 unrouted)
  Top 0.2: SW1.2 6.32,47.45 v6.6,47.17
  Top 0.203: A1.23 39.21,19.37 | R14.1 v6.6,47.17
  Top 0.254: 39.21,19.37 v39.22,19.36 | 6.53,47.09 v6.6,47.17 6.1,46.66 C17.1
  Bottom 0.2: 30.48,23.04 30.2,23.32 30.2,32.03 29.18,33.05 22.25,33.05 17.88,37.41 | 17.88,37.44 17.88,41.1 13.31,45.67 7.7,45.67 7.32,45.29 6.63,45.29 6.5,45.41
  Bottom 0.203: v39.22,19.36 39.22,20.42 37.16,22.48 31.04,22.48 30.48,23.04 | 6.5,45.41 6.24,45.68 6.24,46.6 6.55,46.91 v6.6,47.17
N$20
  Top 0.254: 7.97,38.31 7.78,38.37 IC4.4 7.76,36.71 7.55,36.71 7.55,38.31 | 7.97,38.31 L4.1 | 7.97,36.71 7.97,38.31
N$21
  Top 0.254: A1.39 55.41,32.97 R6.1
N$24
  Top 0.2: R8.2 57.91,38.41 LED4.C
N$25
  Top 0.254: A1.41 R7.1
N$26
  Top 0.2: IC2.6 62.68,45.67 63.07,45.28 63.07,32.35 61.74,31.02 61.74,28.3 59.77,26.33 57.41,26.33 56.35,25.28 A1.35 55.12,25.26
N$27  (via drill 0.4 pad 0.3)
  Top 0.254: C21.1 19.83,12.06 R9.1 20.59,12.06 20.4,12.06
  Top 0.9: 20.4,12.06 17.5,12.06 15.82,13.74 13.66,13.74 12.39,12.47 v12.39,11.53
  Bottom 0.9: v12.39,11.53 12.39,10.9 10.85,9.35 10.85,9.31 X1.2
N$28  (1 unrouted)
  Bottom 0.254: PCB1.I/OREF 32.36,4.42 34.24,4.42 37.64,7.82 37.64,9.45 37.06,10.03 34.49,10.03 34.14,10.39 34.14,11.61 33.76,11.99 31.19,11.99 31.04,11.84
N$29
  pour Top (isolate 0.2): 46.51,10.77 59.78,16.71 59.45,4.25 46.51,4.53
N$31  (via drill 0.4)
  Top 0.2: v53.18,37.9 53.21,37.65 53.21,37.5 53.21,32.1 52.05,30.94 52.05,28.04 52.81,27.28 52.93,27.28 54.18,27.28 A1.36 | IC3.6 59.01,46.51 59.68,45.84 59.68,45.2 59.23,44.75 58.15,44.75 v57.89,45.03
  Bottom 0.2: v57.89,45.03 57.35,44.49 57.3,44.49 54.4,44.49 53.19,43.28 53.18,43.28 v53.18,37.9
N$33
  Top 0.254: 60.55,15.29 63.86,15.29 ANT1.FEED | R19.1 58.3,12.78 58.31,12.78 C4.1
  Top 1: 60.55,15.29 arc90 58.3,13.03 58.31,12.78 58.31,12.65
N$35
  Top 0.254: 49.21,8.06 49.21,8.13 49.23,8.15 49.23,7.85 R4.2
  Top 1: A1.26 49.21,8.06
N$36
  Top 0.406: 26.9,25.3 27.08,25.3 27.13,25.25 27.28,25.25 A1.11
  Top 0.95: 26.9,25.3 24.92,25.3 24.51,25.7 23.57,25.7 20.7,22.84 16.48,22.84 X2.6
N$37
  Top 0.95: A1.10 25.02,27.28 24.64,26.9 23.04,26.9 20.17,24.03 16.51,24.03 X2.4
N$38
  Top 0.406: 26.92,29.26 27.43,29.26 27.46,29.23 27.35,29.23 A1.9
  Top 0.61: 15.01,25.98 17.45,25.98 17.48,26.01
  Top 0.95: 26.92,29.26 25.2,29.26 24.82,29.64 22.23,29.64 19.23,26.64 18.11,26.64 17.48,26.01 | X2.3 15.01,25.98
N$39
  Top 0.406: 26.9,31.27 27.3,31.27 A1.8
  Top 0.95: 26.9,31.27 25.09,31.27 24.69,30.86 21.74,30.86 18.72,27.84 18.09,27.84 17.22,28.7 13.46,28.7 X2.1
RESET  (via drill 0.4)  (2 unrouted)
  Top 0.2: C1.1 57.2,22.5 v57.64,22.94
  Top 0.203: A1.33 57.02,21.28 | 7.95,46.13 7.91,46.06 v6.99,46.06 6.32,45.4 SW2.2
  Bottom 0.2: 30.68,23.5 30.68,32.23 29.39,33.53 22.45,33.53 18.36,37.62 18.36,41.27 13.51,46.13 7.05,46.13 v6.99,46.06
  Bottom 0.203: v57.64,22.94 31.23,22.94 30.68,23.5
RESET2
  Top 0.254: C23.1 IC5.4
RXD_  (via drill 0.4)
  Top 0.2: IC2.4 61.32,45.17 61.32,44.79 61.13,44.6 60.64,44.6 59.72,43.68 58.73,43.68 v58.49,43.43 56.33,41.27 A1.43
  Bottom 0.2: v58.49,43.43 61.18,40.74 SV2.4
SCK  (via drill 0.4)
  Top 0.254: IC1.12 21.88,38.54 v21.67,38.33
  Bottom 0.2: 43.89,38.66 22,38.66 v21.67,38.33
  Bottom 0.254: PCB1.SCK 63.6,27.94 62.94,28.6 53.95,28.6 43.89,38.66
SCK_
  Top 0.203: 27.28,37.3 A1.5 27.19,37.39 27.03,37.39 25.88,38.54 IC1.3
SS  (via drill 0.4)
  Top 0.2: IC1.13 22.57,38.04 22.05,37.52 20.57,37.52 v19.89,38.2
  Bottom 0.2: J1.1 36.56,42.22 36.17,42.22 35.28,43.1 21.41,43.1 19.89,41.58 v19.89,38.2
SS_  (via drill 0.4)
  Top 0.254: v53.02,28.33 53.02,30.42 53.86,31.28 A1.38 | IC1.2 25.54,38.04 25.65,37.94 v25.67,37.5
  Bottom 0.2: v53.02,28.33 53.02,28.69 43.66,38.09
  Bottom 0.254: 43.66,38.09 26.32,38.09 v25.67,37.5
TXD_
  Top 0.2: 55.6,43.16 55.23,43.16 A1.44 54.77,43.28 53.87,42.38 53.87,40.67 54.26,40.28 56.51,40.28 59.25,43.02 61.12,43.02 SV2.5 62.17,44.07 IC2.5
V+  (via drill 0.4)
  Top 0.203: IC2.3 61.17,45.67 60.75,45.26 C8.1 59.52,44.3 58.27,44.3 58.17,44.2 57.56,44.2 57.2,44.55 57.2,44.7 57.07,44.83 57.07,45.29 56.57,45.8 56.57,46.21 C18.1 arc-90 56.52,46.51 IC3.3 IC3.4 IC3.3 | IC1.1 24.3,37.1 C6.1
  Top 0.254: 24.7,36.7 C6.1 | R14.2 R1.2 | C18.1 55.7,46.38 v55.52,46.56 | R1.2 8.89,47.04 8.91,47.07 8.97,47.07 | R1.2 8.89,46.99 8.97,47.07 | 8.97,47.07 9.65,47.07 v9.78,46.94 | IC1.1 24.3,37.09 24.64,36.75 24,36.75 23.75,36.5 23.75,35.28 23.37,34.9 19.84,34.9 18.97,35.76 18.97,38.3 18.31,38.96 17.83,38.96 | 17.83,38.96 C15.1 16.78,38.99 C24.1 16.46,39.22 16.71,38.96 17.8,38.96 17.83,38.99 18.31,38.99 19,39.67 19,43.03 v20.27,44.3 28.91,44.3 29.87,45.26 29.87,46.33 v29.9,46.35 | 17.83,38.96 17.83,37.87 IC5.5
  Bottom 0.254: v55.52,46.56 30.43,46.56 v29.9,46.35 | v9.78,46.94 13.46,46.94 16.1,44.3 v20.27,44.3
VEE
  Top 0.254: A1.52 31.21,45.08 29.84,43.71 29.84,35.48 28.68,34.31 25.35,34.31 24.43,33.4 19.46,33.4 18.8,32.74 18.8,31.79 C16.1 15.6,31.76 14.05,30.2 12.83,30.2 11.94,29.31 11.94,27.28 | 11.94,27.28 11.94,24.79 X2.5 | X2.2 11.96,27.25 11.94,27.28
VPP  (via drill 0.4)  (4 unrouted)
  Top 0.2: IC2.7 62.7,46.17 v63,46.47 63.79,46.47 C9.1 | IC3.7 58.81,47.01 C19.1 59.7,47.16 v59.99,47.45
  Top 0.203: IC3.1 57.39,48.25 56.92,48.72 55.19,48.72 54.84,48.37 | v54.84,48.38 54.84,48.37 | 54.84,48.37 54.84,48.36
  Top 0.254: IC1.14 23.8,37.29 23.24,36.72 22.86,36.72 | v31.64,25.25 31.64,14.78 v30.47,13.62 | v21.03,36.72 22.86,36.72 | C7.1 22.86,36.72
  Bottom 0.203: 54.84,47.37 55.3,47.37 | v54.84,48.39 54.84,47.4
  Bottom 0.254: v63,46.47 62.02,47.45 v59.99,47.45 58.89,46.34 56.91,46.34 55.88,47.37 55.3,47.37 27.24,47.37 23.55,43.68 21.19,43.68 19.32,41.77 19.32,38.81 19.07,38.56 19.07,37.8 19.53,37.34 20.41,37.34 v21.03,36.72 21.26,36.96 23.29,36.96 24.71,35.53 24.71,35.2 25.6,34.31 29.74,34.31 31.64,32.44 v31.64,25.25 | J5.2 30.47,13.49 v30.47,13.62
(copper drawn outside any net)
  shapes: Top area x1

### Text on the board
Top: Reference Designs ARE PROVIDED "AS IS" AND "WITH ALL FAULTS. Arduino LLC DISCLAIMS ALL OTHER WARRANTIES, EXPRESS OR IMPLIED, / REGARDING PRODUCTS, INCLUDING BUT NOT LIMITED TO, ANY IMPLIED WARRANTIES OF MERCHANTABILITY OR FITNESS FOR A / PARTICULAR PURPOSE / Arduino LLC may make changes to specifications and product descriptions at any time, without notice. The Customer must not / rely on the absence or characteristics of any features or instructions marked "reserved" or "undefined." Arduino LLC reserves / these for future definition and shall have no responsibility whatsoever for conflicts or incompatibilities arising from future changes to them. / The product information on the Web Site or Materials is subject to change without notice. Do not finalize a design with this information.
tNames: SW1 | X4 | X5 | IC3 | IC2 | SW2 | L4 | IC1 | IC4 | X3 | X2 | ANT1 | X1 | X6 | X7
